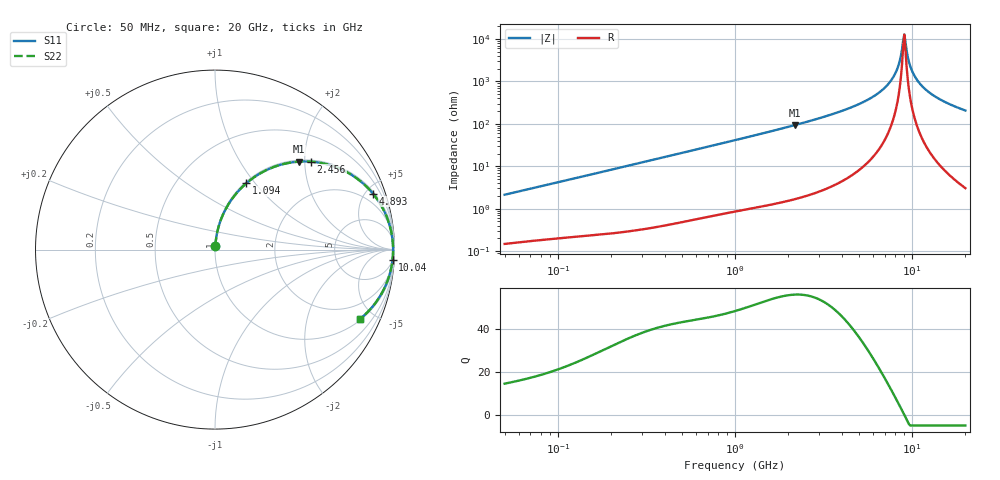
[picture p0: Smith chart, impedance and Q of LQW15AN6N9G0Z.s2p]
!Murata Part Number: LQW15AN6N9G0Z
!These Parameters are Measured in Series Mode Connection
!  o--[Z]--o
!Port1  Port2
!  o-------o
!Freq. Start=50[MHz] Stop=20[GHz], 401[Steps]
# Hz S RI R 50
!Freq.(Hz) S11(Real) S11(Imag) S21(Real) S21(Imag) S12(Real) S12(Imag) S22(Real) S22(Imag)
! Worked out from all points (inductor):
!   401 points, 50 MHz to 20 GHz, reference 50 ohm
!   read as one part in series: L = 6.74 nH near 51.52 MHz
!   highest Q = 55.8 at 2.179 GHz (marker M1), where L = 6.84 nH
!   self-resonance near 8.907 GHz
!   S11 on the Smith chart (normalised r, x): 50 MHz: 1.00, +0.04; 1.094 GHz: 1.02, +0.90; 2.456 GHz: 1.04, +2.14; 4.893 GHz: 1.15, +5.59; 10.04 GHz: 5, -34; 20 GHz: 1.06, -4.13
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5e7  0.00193 0.0212  0.9981 -0.0212  0.9981 -0.0212  0.00193 0.0212
1.364002e8  0.00543 0.0564  0.9946 -0.0564  0.9946 -0.0564  0.00543 0.0564
3.721004e8  0.0266 0.149  0.9734 -0.149  0.9734 -0.149  0.0266 0.149
1e9  0.1505 0.3474  0.8495 -0.3474  0.8495 -0.3474  0.1505 0.3474
1.094034e9  0.1746 0.3695  0.8254 -0.3695  0.8254 -0.3695  0.1746 0.3695
2.179053e9  0.4676 0.4901  0.5324 -0.4901  0.5324 -0.4901  0.4676 0.4901
2.456456e9  0.5343 0.4899  0.4657 -0.4899  0.4657 -0.4899  0.5343 0.4899
2.728004e9  0.5938 0.4821  0.4062 -0.4821  0.4062 -0.4821  0.5938 0.4821
4.89267e9  0.88 0.3118  0.12 -0.3118  0.12 -0.3118  0.88 0.3118
6.311513e9  0.9537 0.1899  0.0463 -0.1899  0.0463 -0.1899  0.9537 0.1899
7.442007e9  0.9809 0.1039  0.0191 -0.1039  0.0191 -0.1039  0.9809 0.1039
8.264682e9  0.9898 0.0478  0.0102 -0.0478  0.0102 -0.0478  0.9898 0.0478
8.516016e9  0.9912 0.0316  0.00882 -0.0316  0.00882 -0.0316  0.9912 0.0316
8.774992e9  0.992 0.0154  0.008 -0.0154  0.008 -0.0154  0.992 0.0154
9.041845e9  0.9923 -0.000753  0.00771 0.000753  0.00771 0.000753  0.9923 -0.000753
9.178299e9  0.9922 -0.00885  0.00777 0.00885  0.00777 0.00885  0.9922 -0.00885
9.600142e9  0.9913 -0.0331  0.00873 0.0331  0.00873 0.0331  0.9913 -0.0331
1.004137e10  0.9891 -0.0574  0.0109 0.0574  0.0109 0.0574  0.9891 -0.0574
1.098561e10  0.9812 -0.1055  0.0188 0.1055  0.0188 0.1055  0.9812 -0.1055
1.276073e10  0.9573 -0.1841  0.0427 0.1841  0.0427 0.1841  0.9573 -0.1841
1.573793e10  0.9012 -0.2873  0.0988 0.2873  0.0988 0.2873  0.9012 -0.2873
2e10  0.8065 -0.3877  0.1935 0.3877  0.1935 0.3877  0.8065 -0.3877
